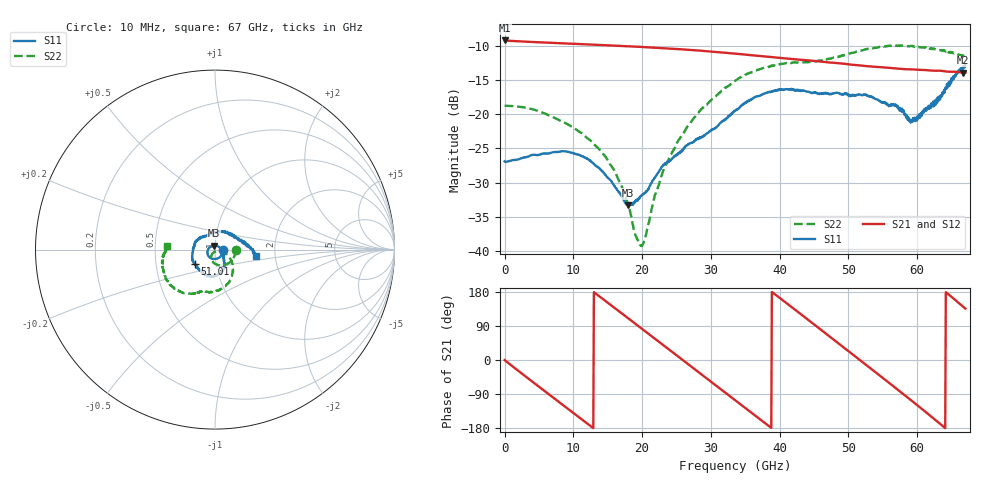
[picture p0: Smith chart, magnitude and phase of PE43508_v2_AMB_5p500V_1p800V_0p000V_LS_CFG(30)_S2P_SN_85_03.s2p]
!Keysight Technologies,N5227A,US51270237,A.10.43.00
!Date: Wednesday, August 22, 2018 17:09:41
!Correction: S11(Full 2 Port(1,3))
!S31(Full 2 Port(1,3))
!S13(Full 2 Port(1,3))
!S33(Full 2 Port(1,3))
!S2P File: Measurements: S11, S31, S13, S33:
# Hz S  dB  R 50
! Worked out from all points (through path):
!   801 points, 10 MHz to 67 GHz, reference 50 ohm
!   highest |S21| = -9.20 dB at 10 MHz (marker M1); lowest = -13.9 dB at 66.67 GHz (marker M2)
!   group delay of S21, straight-line fit = 38.9 ps
!   lowest |S11| = -33.3 dB at 17.93 GHz (marker M3), VSWR 1.04, Z = 49.6 + j2.1 ohm
!   |S11| at or under -10 dB: start of sweep to end of sweep
!   |S22| runs from -39.3 to -9.9 dB; largest |S21 - S12| = 0.0021
!   S11 on the Smith chart (normalised r, x): 10 MHz: 1.09, -0.00; 51.01 GHz: 0.79, -0.13; 67 GHz: 1.59, -0.12
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1e7  -26.90 -0.7  -9.20 -0.2  -9.20 -0.2  -18.74 -0.4
2.522125e9  -26.42 -38.2  -9.34 -35.9  -9.34 -35.9  -18.95 -25.9
5.787888e9  -25.77 -80.9  -9.49 -81.4  -9.49 -81.4  -19.86 -56.0
8.300012e9  -25.43 -111.5  -9.61 -116.2  -9.61 -116.2  -21.05 -76.9
1.123082e10  -26.12 -143.9  -9.74 -156.7  -9.74 -156.7  -22.78 -97.3
1.483154e10  -29.12 169.6  -9.90 153.5  -9.90 153.6  -26.49 -116.7
1.792982e10  -33.35 99.9  -10.05 110.7  -10.04 110.7  -33.10 -120.2
1.910215e10  -32.77 65.7  -10.11 94.5  -10.11 94.5  -37.86 -102.1
1.993952e10  -31.81 45.4  -10.15 82.8  -10.15 82.9  -39.31 -62.6
2.236791e10  -28.50 -2.4  -10.29 49.2  -10.29 49.2  -30.47 -17.5
2.722469e10  -24.21 -40.2  -10.60 -18.4  -10.60 -18.3  -20.96 -28.4
3.049045e10  -22.06 -50.1  -10.87 -63.9  -10.86 -63.8  -17.56 -42.1
3.3505e10  -19.50 -61.7  -11.13 -105.9  -11.12 -105.9  -15.12 -57.7
3.88642e10  -16.74 -90.8  -11.63 179.7  -11.64 179.7  -12.94 -84.1
4.472582e10  -16.85 -119.9  -12.16 97.8  -12.15 97.8  -12.34 -105.3
4.75729e10  -16.98 -128.9  -12.44 57.7  -12.44 57.5  -11.78 -111.8
5.100614e10  -17.23 -143.6  -12.79 9.2  -12.78 9.1  -10.91 -121.0
5.586291e10  -18.82 168.3  -13.20 -59.7  -13.20 -60.0  -9.98 -140.4
5.96311e10  -20.50 100.1  -13.46 -113.8  -13.49 -114.0  -10.14 -155.6
6.331555e10  -17.86 30.9  -13.63 -168.4  -13.68 -168.7  -10.62 -170.8
6.666505e10  -13.39 -5.6  -13.91 140.8  -13.97 141.1  -11.41 178.4
6.7e10  -12.67 -8.6  -13.91 135.6  -13.97 135.8  -11.48 176.2
